| IBIS file stm32h563_573_wlcsp80-smps.ibs
[IBIS ver] 4.2
[File name] stm32h563_573_wlcsp80-smps.ibs
[File Rev] 1.1
[Date] 07-05-2024
[Source] Data Created at STMicroelectronics
[Notes]  File originated from ELDO simulations.
[Disclaimer]  This information is for modeling purpose only and is
   not guaranteed. The information is subject to change without
   notice.
[Copyright] Copyright 2024 STMicroelectronics Inc.
|   Component stm32h563_573_wlcsp80-smps
[Component] stm32h563_573_wlcsp80-smps
[Manufacturer] STMicroelectronics
[Package]
| variable   typ   min   max
R_pkg  0  NA  NA
L_pkg  0  NA  NA
C_pkg  0  NA  NA
[Pin]   signal_name   model_name
A1  VDD  power
A3  PD0  io8_ft_i3c_spi
A5  PD2  io8_ft_i3c_spi
A7  VDD  power
A9  VCAP  nc
B2  VDDUSB  power
B4  PD1  io8_ft_i3c_spi
B6  PB4  io8_ft_i3c_spi
B8  VSS  gnd
B10  VBAT  power
C1  PA12  io8usb_ft_i3c_spi_phy
C3  PC10  io8_ft_i3c_spi
C5  PB3  io8_ft_i3c_spi
C7  PB7  io8_ft_i3c_spi
C9  PC13  io8_ft_i3c_spi
D2  VSS  gnd
D4  PA15  io8_ft_i3c_spi
D6  PB5  io8_ft_i3c_spi
D8  BOOT0  vpphv
D10  PC14-OSC32_IN  io8_ft_i3c_spi
E1  PA11  io8usb_ft_i3c_spi_phy
E3  PA14  io8_ft_i3c_spi
E5  PC11  io8_ft_i3c_spi
E7  PB6  io8_ft_i3c_spi
E9  PB8  io8_ft_i3c_spi
F2  PC9  io8_ft_i3c_spi
F4  PA13  io8_ft_i3c_spi
F6  PC12  io8_ft_i3c_spi
F8  NRST  ioreset_ft_v33
F10  PC15-OSC32_OUT  io8_ft_i3c_spi
G1  VDD  power
G3  PA8  io8_ft_i3c_spi
G5  PA10  io8_ft_i3c_spi
G7  PC1  io8_ft_spi
G9  VSS  gnd
H2  VSS  gnd
H4  PA9  io8_ft_i3c_spi
H6  PA6  io8_ft_spi
H8  PC0  io8_ft_spi
H10  VDD  power
J1  PD15  io8_ft_i3c_spi
J3  PC6  io8_ft_i3c_spi
J5  PC8  io8_ft_i3c_spi
J7  PA1  io8_ft_spi_tamp
J9  PH1-OSC_OUT  io8_ft_i3c_spi
K2  PD14  io8_ft_i3c_spi
K4  PC7  io8_ft_i3c_spi
K6  PA7  io8_ft_spi
K8  PA0  io8_ft_spi
K10  PH0-OSC_IN  io8_ft_i3c_spi
L1  PB15  io8_ft_spi
L3  PB12  io8_ft_i3c_spi
L5  PB2  io8_ft_i3c_spi
L7  PA5  io8_ft_spi
L9  PC3  io8_ft_spi
|M2  PB13  io8usb_ft_pd
M2  PB13  nc
M4  PE10  io8_ft_i3c_spi
M6  PC4  io8_ft_spi
M8  PA2  io8_ft_spi
M10  PC2  io8_ft_spi
|N1  PB14  io8usb_ft_pd
N1  PB14  nc
N3  VSSSMPS  nc
N5  PE8  io8_ft_i3c_spi
N7  PC5  io8_ft_spi
N9  VSSA  nc
P2  VSS  gnd
P4  PB10  io8_ft_i3c_spi
P6  PB1  io8_ft_spi
P8  VSS  gnd
P10  VDDA  nc
R1  VDD  power
R3  VDDSMPS  nc
R5  PE9  io8_ft_i3c_spi
R7  PB0  io8_ft_spi
R9  PA4  io8_ft_spi
T2  VCAP  nc
T4  VLXSMPS  nc
T6  PE7  io8_ft_i3c_spi
T8  VDD  power
T10  PA3  io8_ft_spi
[Package Model]   484-wlcsp-25-221014
[Pin Mapping]   pulldown_ref   pullup_ref   | Comment
A1  nc  vddiom
A3  gndio  vddiom
A5  gndio  vddiom
A7  nc  vddiom
A9  nc  nc
B2  nc  vddusb
B4  gndio  vddiom
B6  gndio  vddiom
B8  gndio  nc
B10  nc  vsw
C1  gndio  vddiom  | Depending on IO usage
| C1  gndio  vddusb  | Depending on IO usage
C3  gndio  vddiom
C5  gndio  vddiom
C7  gndio  vddiom
C9  gndio  vddiom  | Depending on IO usage
| C9  gndio  vsw  | Depending on IO usage
D2  gndio  nc
D4  gndio  vddiom
D6  gndio  vddiom
D8  gndio  vddiom
D10  gndio  vddiom  | Depending on IO usage
| D10  gndio  vsw  | Depending on IO usage
E1  gndio  vddiom  | Depending on IO usage
| E1  gndio  vddusb  | Depending on IO usage
E3  gndio  vddiom
E5  gndio  vddiom
E7  gndio  vddiom
E9  gndio  vddiom
F2  gndio  vddiom
F4  gndio  vddiom  | Depending on IO usage
| F4  gndio  vddusb  | Depending on IO usage
F6  gndio  vddiom
F8  gndio  vddiom
F10  gndio  vddiom  | Depending on IO usage
| F10  gndio  vsw  | Depending on IO usage
G1  nc  vddiom
G3  gndio  vddiom
G5  gndio  vddiom  | Depending on IO usage
| G5  gndio  vddusb  | Depending on IO usage
G7  gndio  vddiom
G9  gndio  nc
H2  gndio  nc
H4  gndio  vddiom  | Depending on IO usage
| H4  gndio  vddusb  | Depending on IO usage
H6  gndio  vddiom
H8  gndio  vddiom
H10  nc  vddiom
J1  gndio  vddiom
J3  gndio  vddiom
J5  gndio  vddiom
J7  gndio  vddiom
J9  gndio  vddiom
K2  gndio  vddiom
K4  gndio  vddiom
K6  gndio  vddiom
K8  gndio  vddiom
K10  gndio  vddiom
L1  gndio  vddiom
L3  gndio  vddiom
L5  gndio  vddiom
L7  gndio  vddiom
L9  gndio  vddiom
|M2  gndio  vddiom
M2  nc nc
M4  gndio  vddiom
M6  gndio  vddiom
M8  gndio  vddiom
M10  gndio  vddiom
|N1  gndio  vddiom
N1  nc nc
N3  nc  nc
N5  gndio  vddiom
N7  gndio  vddiom
N9  nc  nc
P2  gndio  nc
P4  gndio  vddiom
P6  gndio  vddiom
P8  gndio  nc
P10  nc  nc
R1  nc  vddiom
R3  nc  nc
R5  gndio  vddiom
R7  gndio  vddiom
R9  gndio  vddiom
T2  nc  nc
T4  nc  nc
T6  gndio  vddiom
T8  nc  vddiom
T10  gndio  vddiom
[Model Selector] io8_ft_i3c_spi
io8_ft_spi_ls_1v2 "io8_ft spi low speed @ 1.2V"
io8_ft_spi_ls_1v8 "io8_ft spi low speed @ 1.8V"
io8_ft_spi_ls_3v3 "io8_ft spi low speed @ 3.3V"
io8_ft_spi_ms_1v2 "io8_ft spi med speed @ 1.2V"
io8_ft_spi_ms_1v8 "io8_ft spi med speed @ 1.8V"
io8_ft_spi_ms_3v3 "io8_ft spi med speed @ 3.3V"
io8_ft_spi_fs_1v2 "io8_ft spi fast speed @ 1.2V"
io8_ft_spi_fs_1v8 "io8_ft spi fast speed @ 1.8V"
io8_ft_spi_fs_3v3 "io8_ft spi fast speed @ 3.3V"
io8_ft_spi_hs_1v2 "io8_ft spi high speed @ 1.2V"
io8_ft_spi_hs_1v8 "io8_ft spi high speed @ 1.8V"
io8_ft_spi_hs_3v3 "io8_ft spi high speed @ 3.3V"
io8_ft_hslv_spi_ls_1v2 "io8_ft spi hslv low speed @ 1.2V"
io8_ft_hslv_spi_ls_1v8 "io8_ft spi hslv low speed @ 1.8V"
io8_ft_hslv_spi_ls_2v5 "io8_ft spi hslv low speed @ 2.5V"
io8_ft_hslv_spi_ms_1v2 "io8_ft spi hslv med speed @ 1.2V"
io8_ft_hslv_spi_ms_1v8 "io8_ft spi hslv med speed @ 1.8V"
io8_ft_hslv_spi_ms_2v5 "io8_ft spi hslv med speed @ 2.5V"
io8_ft_hslv_spi_fs_1v2 "io8_ft spi hslv fast speed @ 1.2V"
io8_ft_hslv_spi_fs_1v8 "io8_ft spi hslv fast speed @ 1.8V"
io8_ft_hslv_spi_fs_2v5 "io8_ft spi hslv fast speed @ 2.5V"
io8_ft_hslv_spi_hs_1v2 "io8_ft spi hslv high speed @ 1.2V"
io8_ft_hslv_spi_hs_1v8 "io8_ft spi hslv high speed @ 1.8V"
io8_ft_hslv_spi_hs_2v5 "io8_ft spi hslv high speed @ 2.5V"
io8_ft_i3c_spi_ls_1v2 "io8_ft i3c spi open-drain low speed @ 1.2V"
io8_ft_i3c_spi_ls_1v8 "io8_ft i3c spi open-drain low speed @ 1.8V"
io8_ft_i3c_spi_ls_3v3 "io8_ft i3c spi open-drain low speed @ 3.3V"
io8_ft_i3c_spi_ms_1v2 "io8_ft i3c spi open-drain med speed @ 1.2V"
io8_ft_i3c_spi_ms_1v8 "io8_ft i3c spi open-drain med speed @ 1.8V"
io8_ft_i3c_spi_ms_3v3 "io8_ft i3c spi open-drain med speed @ 3.3V"
io8_ft_i3c_spi_fs_1v2 "io8_ft i3c spi open-drain fast speed @ 1.2V"
io8_ft_i3c_spi_fs_1v8 "io8_ft i3c spi open-drain fast speed @ 1.8V"
io8_ft_i3c_spi_fs_3v3 "io8_ft i3c spi open-drain fast speed @ 3.3V"
io8_ft_i3c_spi_hs_1v2 "io8_ft i3c spi open-drain high speed @ 1.2V"
io8_ft_i3c_spi_hs_1v8 "io8_ft i3c spi open-drain high speed @ 1.8V"
io8_ft_i3c_spi_hs_3v3 "io8_ft i3c spi open-drain high speed @ 3.3V"
io8_ft_hslv_i3c_spi_ls_1v2 "io8_ft hslv i3c spi open-drain low speed @ 1.2V"
io8_ft_hslv_i3c_spi_ls_1v8 "io8_ft hslv i3c spi open-drain low speed @ 1.8V"
io8_ft_hslv_i3c_spi_ls_2v5 "io8_ft hslv i3c spi open-drain low speed @ 2.5V"
io8_ft_hslv_i3c_spi_ms_1v2 "io8_ft hslv i3c spi open-drain med speed @ 1.2V"
io8_ft_hslv_i3c_spi_ms_1v8 "io8_ft hslv i3c spi open-drain med speed @ 1.8V"
io8_ft_hslv_i3c_spi_ms_2v5 "io8_ft hslv i3c spi open-drain med speed @ 2.5V"
io8_ft_hslv_i3c_spi_fs_1v2 "io8_ft hslv i3c spi open-drain fast speed @ 1.2V"
io8_ft_hslv_i3c_spi_fs_1v8 "io8_ft hslv i3c spi open-drain fast speed @ 1.8V"
io8_ft_hslv_i3c_spi_fs_2v5 "io8_ft hslv i3c spi open-drain fast speed @ 2.5V"
io8_ft_hslv_i3c_spi_hs_1v2 "io8_ft hslv i3c spi open-drain high speed @ 1.2V"
io8_ft_hslv_i3c_spi_hs_1v8 "io8_ft hslv i3c spi open-drain high speed @ 1.8V"
io8_ft_hslv_i3c_spi_hs_2v5 "io8_ft hslv i3c spi open-drain high speed @ 2.5V"
io8_ft_i3c_fmp_spi_3v3 "io8_ft i3c fm+ spi open-drain @ 3.3V"
io8_ft_i3c_fmp_spi_1v8 "io8_ft i3c fm+ spi open-drain @ 1.8V"
io8_ft_i3c_fmp_spi_1v2 "io8_ft i3c fm+ spi open-drain @ 1.2V"
[Model Selector] io8_ft_spi
io8_ft_spi_ls_1v2 "io8_ft spi low speed @ 1.2V"
io8_ft_spi_ls_1v8 "io8_ft spi low speed @ 1.8V"
io8_ft_spi_ls_3v3 "io8_ft spi low speed @ 3.3V"
io8_ft_spi_ms_1v2 "io8_ft spi med speed @ 1.2V"
io8_ft_spi_ms_1v8 "io8_ft spi med speed @ 1.8V"
io8_ft_spi_ms_3v3 "io8_ft spi med speed @ 3.3V"
io8_ft_spi_fs_1v2 "io8_ft spi fast speed @ 1.2V"
io8_ft_spi_fs_1v8 "io8_ft spi fast speed @ 1.8V"
io8_ft_spi_fs_3v3 "io8_ft spi fast speed @ 3.3V"
io8_ft_spi_hs_1v2 "io8_ft spi high speed @ 1.2V"
io8_ft_spi_hs_1v8 "io8_ft spi high speed @ 1.8V"
io8_ft_spi_hs_3v3 "io8_ft spi high speed @ 3.3V"
io8_ft_hslv_spi_ls_1v2 "io8_ft spi hslv low speed @ 1.2V"
io8_ft_hslv_spi_ls_1v8 "io8_ft spi hslv low speed @ 1.8V"
io8_ft_hslv_spi_ls_2v5 "io8_ft spi hslv low speed @ 2.5V"
io8_ft_hslv_spi_ms_1v2 "io8_ft spi hslv med speed @ 1.2V"
io8_ft_hslv_spi_ms_1v8 "io8_ft spi hslv med speed @ 1.8V"
io8_ft_hslv_spi_ms_2v5 "io8_ft spi hslv med speed @ 2.5V"
io8_ft_hslv_spi_fs_1v2 "io8_ft spi hslv fast speed @ 1.2V"
io8_ft_hslv_spi_fs_1v8 "io8_ft spi hslv fast speed @ 1.8V"
io8_ft_hslv_spi_fs_2v5 "io8_ft spi hslv fast speed @ 2.5V"
io8_ft_hslv_spi_hs_1v2 "io8_ft spi hslv high speed @ 1.2V"
io8_ft_hslv_spi_hs_1v8 "io8_ft spi hslv high speed @ 1.8V"
io8_ft_hslv_spi_hs_2v5 "io8_ft spi hslv high speed @ 2.5V"
[Model Selector] io8_ft_spi_tamp
io8_ft_spi_ls_1v2 "io8_ft spi low speed @ 1.2V"
io8_ft_spi_ls_1v8 "io8_ft spi low speed @ 1.8V"
io8_ft_spi_ls_3v3 "io8_ft spi low speed @ 3.3V"
io8_ft_spi_ms_1v2 "io8_ft spi med speed @ 1.2V"
io8_ft_spi_ms_1v8 "io8_ft spi med speed @ 1.8V"
io8_ft_spi_ms_3v3 "io8_ft spi med speed @ 3.3V"
io8_ft_spi_fs_1v2 "io8_ft spi fast speed @ 1.2V"
io8_ft_spi_fs_1v8 "io8_ft spi fast speed @ 1.8V"
io8_ft_spi_fs_3v3 "io8_ft spi fast speed @ 3.3V"
io8_ft_spi_hs_1v2 "io8_ft spi high speed @ 1.2V"
io8_ft_spi_hs_1v8 "io8_ft spi high speed @ 1.8V"
io8_ft_spi_hs_3v3 "io8_ft spi high speed @ 3.3V"
io8_ft_hslv_spi_ls_1v2 "io8_ft spi hslv low speed @ 1.2V"
io8_ft_hslv_spi_ls_1v8 "io8_ft spi hslv low speed @ 1.8V"
io8_ft_hslv_spi_ls_2v5 "io8_ft spi hslv low speed @ 2.5V"
io8_ft_hslv_spi_ms_1v2 "io8_ft spi hslv med speed @ 1.2V"
io8_ft_hslv_spi_ms_1v8 "io8_ft spi hslv med speed @ 1.8V"
io8_ft_hslv_spi_ms_2v5 "io8_ft spi hslv med speed @ 2.5V"
io8_ft_hslv_spi_fs_1v2 "io8_ft spi hslv fast speed @ 1.2V"
io8_ft_hslv_spi_fs_1v8 "io8_ft spi hslv fast speed @ 1.8V"
io8_ft_hslv_spi_fs_2v5 "io8_ft spi hslv fast speed @ 2.5V"
io8_ft_hslv_spi_hs_1v2 "io8_ft spi hslv high speed @ 1.2V"
io8_ft_hslv_spi_hs_1v8 "io8_ft spi hslv high speed @ 1.8V"
io8_ft_hslv_spi_hs_2v5 "io8_ft spi hslv high speed @ 2.5V"
io8_ft_tamp_v33_1v2 "io8_ft tamp V33 @ 1.2V"
io8_ft_tamp_v33_1v8 "io8_ft tamp V33 @ 1.2V"
io8_ft_tamp_v33_3v3 "io8_ft tamp V33 @ 1.2V"
[Model Selector] io8usb_ft_i3c_spi_phy
io8_ft_spi_ls_1v2 "io8_ft spi low speed @ 1.2V"
io8_ft_spi_ls_1v8 "io8_ft spi low speed @ 1.8V"
io8_ft_spi_ls_3v3 "io8_ft spi low speed @ 3.3V"
io8_ft_spi_ms_1v2 "io8_ft spi med speed @ 1.2V"
io8_ft_spi_ms_1v8 "io8_ft spi med speed @ 1.8V"
io8_ft_spi_ms_3v3 "io8_ft spi med speed @ 3.3V"
io8_ft_spi_fs_1v2 "io8_ft spi fast speed @ 1.2V"
io8_ft_spi_fs_1v8 "io8_ft spi fast speed @ 1.8V"
io8_ft_spi_fs_3v3 "io8_ft spi fast speed @ 3.3V"
io8_ft_spi_hs_1v2 "io8_ft spi high speed @ 1.2V"
io8_ft_spi_hs_1v8 "io8_ft spi high speed @ 1.8V"
io8_ft_spi_hs_3v3 "io8_ft spi high speed @ 3.3V"
io8_ft_hslv_spi_ls_1v2 "io8_ft spi hslv low speed @ 1.2V"
io8_ft_hslv_spi_ls_1v8 "io8_ft spi hslv low speed @ 1.8V"
io8_ft_hslv_spi_ls_2v5 "io8_ft spi hslv low speed @ 2.5V"
io8_ft_hslv_spi_ms_1v2 "io8_ft spi hslv med speed @ 1.2V"
io8_ft_hslv_spi_ms_1v8 "io8_ft spi hslv med speed @ 1.8V"
io8_ft_hslv_spi_ms_2v5 "io8_ft spi hslv med speed @ 2.5V"
io8_ft_hslv_spi_fs_1v2 "io8_ft spi hslv fast speed @ 1.2V"
io8_ft_hslv_spi_fs_1v8 "io8_ft spi hslv fast speed @ 1.8V"
io8_ft_hslv_spi_fs_2v5 "io8_ft spi hslv fast speed @ 2.5V"
io8_ft_hslv_spi_hs_1v2 "io8_ft spi hslv high speed @ 1.2V"
io8_ft_hslv_spi_hs_1v8 "io8_ft spi hslv high speed @ 1.8V"
io8_ft_hslv_spi_hs_2v5 "io8_ft spi hslv high speed @ 2.5V"
io8_ft_i3c_spi_ls_1v2 "io8_ft i3c spi open-drain low speed @ 1.2V"
io8_ft_i3c_spi_ls_1v8 "io8_ft i3c spi open-drain low speed @ 1.8V"
io8_ft_i3c_spi_ls_3v3 "io8_ft i3c spi open-drain low speed @ 3.3V"
io8_ft_i3c_spi_ms_1v2 "io8_ft i3c spi open-drain med speed @ 1.2V"
io8_ft_i3c_spi_ms_1v8 "io8_ft i3c spi open-drain med speed @ 1.8V"
io8_ft_i3c_spi_ms_3v3 "io8_ft i3c spi open-drain med speed @ 3.3V"
io8_ft_i3c_spi_fs_1v2 "io8_ft i3c spi open-drain fast speed @ 1.2V"
io8_ft_i3c_spi_fs_1v8 "io8_ft i3c spi open-drain fast speed @ 1.8V"
io8_ft_i3c_spi_fs_3v3 "io8_ft i3c spi open-drain fast speed @ 3.3V"
io8_ft_i3c_spi_hs_1v2 "io8_ft i3c spi open-drain high speed @ 1.2V"
io8_ft_i3c_spi_hs_1v8 "io8_ft i3c spi open-drain high speed @ 1.8V"
io8_ft_i3c_spi_hs_3v3 "io8_ft i3c spi open-drain high speed @ 3.3V"
io8_ft_hslv_i3c_spi_ls_1v2 "io8_ft hslv i3c spi open-drain low speed @ 1.2V"
io8_ft_hslv_i3c_spi_ls_1v8 "io8_ft hslv i3c spi open-drain low speed @ 1.8V"
io8_ft_hslv_i3c_spi_ls_2v5 "io8_ft hslv i3c spi open-drain low speed @ 2.5V"
io8_ft_hslv_i3c_spi_ms_1v2 "io8_ft hslv i3c spi open-drain med speed @ 1.2V"
io8_ft_hslv_i3c_spi_ms_1v8 "io8_ft hslv i3c spi open-drain med speed @ 1.8V"
io8_ft_hslv_i3c_spi_ms_2v5 "io8_ft hslv i3c spi open-drain med speed @ 2.5V"
io8_ft_hslv_i3c_spi_fs_1v2 "io8_ft hslv i3c spi open-drain fast speed @ 1.2V"
io8_ft_hslv_i3c_spi_fs_1v8 "io8_ft hslv i3c spi open-drain fast speed @ 1.8V"
io8_ft_hslv_i3c_spi_fs_2v5 "io8_ft hslv i3c spi open-drain fast speed @ 2.5V"
io8_ft_hslv_i3c_spi_hs_1v2 "io8_ft hslv i3c spi open-drain high speed @ 1.2V"
io8_ft_hslv_i3c_spi_hs_1v8 "io8_ft hslv i3c spi open-drain high speed @ 1.8V"
io8_ft_hslv_i3c_spi_hs_2v5 "io8_ft hslv i3c spi open-drain high speed @ 2.5V"
io8_ft_i3c_fmp_spi_3v3 "io8_ft i3c fm+ spi open-drain @ 3.3V"
io8_ft_i3c_fmp_spi_1v8 "io8_ft i3c fm+ spi open-drain @ 1.8V"
io8_ft_i3c_fmp_spi_1v2 "io8_ft i3c fm+ spi open-drain @ 1.2V"
io8usb_ft_phy_ls_2v5 "iousb ft low speed @ 2.5V"
io8usb_ft_phy_ls_3v3 "iousb ft low speed @ 3.3V"
io8usb_ft_phy_fs_2v5 "iousb ft fast speed @ 2.5V"
io8usb_ft_phy_fs_3v3 "iousb ft fast speed @ 3.3V"
[Model Selector] ioreset_ft_v33
ioreset_ft_v33_1v2 "Reset PAD. 5V tolerant. 1.2V range"
ioreset_ft_v33_1v8 "Reset PAD. 5V tolerant. 1.8V range"
ioreset_ft_v33_3v3 "Reset PAD. 5V tolerant. 3.3V range"
[Model Selector] vpphv
vpphv_1v2 "Flash Test cell v33 = 1.2 V range"
vpphv_1v8 "Flash Test cell v33 = 1.8 V range"
vpphv_3v3 "Flash Test cell v33 = 3.3 V range"
[Define Package Model]  484-wlcsp-25-221014
[Manufacturer]  Unknown
[OEM]  Unknown
[Description]  None
[Number Of Pins]  70
[Pin Numbers]
| Pin Num   Terminal Name
D8 | BOOT0
F8 | NRST
K8 | PA0
J7 | PA1
M8 | PA2
T10 | PA3
R9 | PA4
L7 | PA5
H6 | PA6
K6 | PA7
G3 | PA8
H4 | PA9
G5 | PA10
E1 | PA11
C1 | PA12
F4 | PA13
E3 | PA14
D4 | PA15
R7 | PB0
P6 | PB1
L5 | PB2
C5 | PB3
B6 | PB4
D6 | PB5
E7 | PB6
C7 | PB7
E9 | PB8
P4 | PB10
L3 | PB12
M2 | PB13
N1 | PB14
L1 | PB15
H8 | PC0
G7 | PC1
M10 | PC2
L9 | PC3
M6 | PC4
N7 | PC5
J3 | PC6
K4 | PC7
J5 | PC8
F2 | PC9
C3 | PC10
E5 | PC11
F6 | PC12
C9 | PC13
D10 | PC14-OSC32_IN
F10 | PC15-OSC32_OUT
A3 | PD0
B4 | PD1
A5 | PD2
K2 | PD14
J1 | PD15
T6 | PE7
N5 | PE8
R5 | PE9
M4 | PE10
K10 | PH0-OSC_IN
J9 | PH1-OSC_OUT
B10 | VBAT
T2 | VCAP
A9 | VCAP
A1 | VDD
B2 | VDDUSB
P10 | VDDA
R3 | VDDSMPS
T4 | VLXSMPS
B8 | VSS
N9 | VSSA
N3 | VSSSMPS
|[Merged Pins]  A1
|A7  |  VDD
|G1  |  VDD
|H10  |  VDD
|R1  |  VDD
|T8  |  VDD
|[Merged Pins]  B8
|D2  |  VSS
|G9  |  VSS
|H2  |  VSS
|P2  |  VSS
|P8  |  VSS
[Model Data]
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[End Model Data]
[End Package Model]
|End [Component]
| Models and submodels in the file (64): io8_ft_hslv_i3c_spi_fs_1v2 (I/O_open_drain), io8_ft_hslv_i3c_spi_fs_1v8 (I/O_open_drain), io8_ft_hslv_i3c_spi_fs_2v5 (I/O_open_drain), io8_ft_hslv_i3c_spi_hs_1v2 (I/O_open_drain), io8_ft_hslv_i3c_spi_hs_1v8 (I/O_open_drain), io8_ft_hslv_i3c_spi_hs_2v5 (I/O_open_drain), io8_ft_hslv_i3c_spi_ls_1v2 (I/O_open_drain), io8_ft_hslv_i3c_spi_ls_1v8 (I/O_open_drain), io8_ft_hslv_i3c_spi_ls_2v5 (I/O_open_drain), io8_ft_hslv_i3c_spi_ms_1v2 (I/O_open_drain), io8_ft_hslv_i3c_spi_ms_1v8 (I/O_open_drain), io8_ft_hslv_i3c_spi_ms_2v5 (I/O_open_drain), io8_ft_hslv_spi_fs_1v2 (I/O), io8_ft_hslv_spi_fs_1v8 (I/O), io8_ft_hslv_spi_fs_2v5 (I/O), io8_ft_hslv_spi_hs_1v2 (I/O), io8_ft_hslv_spi_hs_1v8 (I/O), io8_ft_hslv_spi_hs_2v5 (I/O), io8_ft_hslv_spi_ls_1v2 (I/O), io8_ft_hslv_spi_ls_1v8 (I/O), io8_ft_hslv_spi_ls_2v5 (I/O), io8_ft_hslv_spi_ms_1v2 (I/O), io8_ft_hslv_spi_ms_1v8 (I/O), io8_ft_hslv_spi_ms_2v5 (I/O), io8_ft_i3c_fmp_spi_1v2 (I/O_open_drain), io8_ft_i3c_fmp_spi_1v8 (I/O_open_drain), io8_ft_i3c_fmp_spi_3v3 (I/O_open_drain), io8_ft_i3c_spi_fs_1v2 (I/O_open_drain), io8_ft_i3c_spi_fs_1v8 (I/O_open_drain), io8_ft_i3c_spi_fs_3v3 (I/O_open_drain), io8_ft_i3c_spi_hs_1v2 (I/O_open_drain), io8_ft_i3c_spi_hs_1v8 (I/O_open_drain), io8_ft_i3c_spi_hs_3v3 (I/O_open_drain), io8_ft_i3c_spi_ls_1v2 (I/O_open_drain), io8_ft_i3c_spi_ls_1v8 (I/O_open_drain), io8_ft_i3c_spi_ls_3v3 (I/O_open_drain), io8_ft_i3c_spi_ms_1v2 (I/O_open_drain), io8_ft_i3c_spi_ms_1v8 (I/O_open_drain), io8_ft_i3c_spi_ms_3v3 (I/O_open_drain), io8_ft_spi_fs_1v2 (I/O), io8_ft_spi_fs_1v8 (I/O), io8_ft_spi_fs_3v3 (I/O), io8_ft_spi_hs_1v2 (I/O), io8_ft_spi_hs_1v8 (I/O), io8_ft_spi_hs_3v3 (I/O), io8_ft_spi_ls_1v2 (I/O), io8_ft_spi_ls_1v8 (I/O), io8_ft_spi_ls_3v3 (I/O), io8_ft_spi_ms_1v2 (I/O), io8_ft_spi_ms_1v8 (I/O), io8_ft_spi_ms_3v3 (I/O), io8_ft_tamp_v33_1v2 (I/O), io8_ft_tamp_v33_1v8 (I/O), io8_ft_tamp_v33_3v3 (I/O), io8usb_ft_phy_fs_2v5 (I/O), io8usb_ft_phy_fs_3v3 (I/O), io8usb_ft_phy_ls_2v5 (I/O), io8usb_ft_phy_ls_3v3 (I/O), ioreset_ft_v33_1v2 (I/O_open_drain), ioreset_ft_v33_1v8 (I/O_open_drain), ioreset_ft_v33_3v3 (I/O_open_drain), vpphv_1v2 (Input), vpphv_1v8 (Input), vpphv_3v3 (Input)
